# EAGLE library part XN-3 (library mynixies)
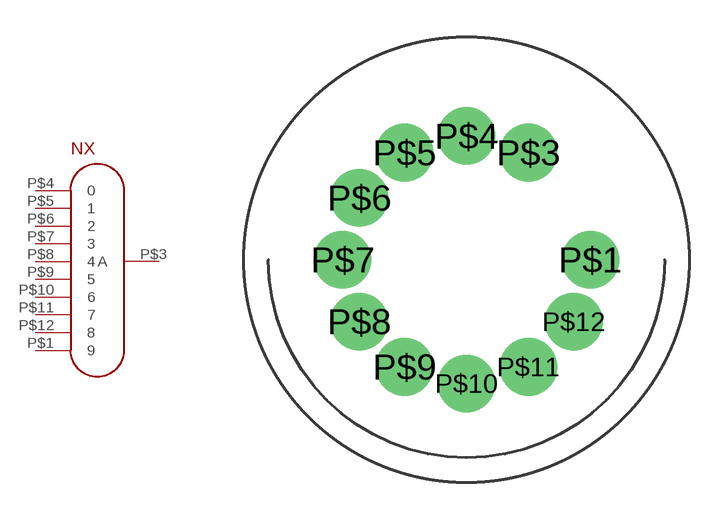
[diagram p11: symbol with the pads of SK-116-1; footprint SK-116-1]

Designator prefix NX

## XN-3  [SK-116-1]
P$1  9
P$3  A
P$4  0
P$5  1
P$6  2
P$7  3
P$8  4
P$9  5
P$10  6
P$11  7
P$12  8

## Footprint SK-116-1 (pad centres in mm)
drill 1.55: P$1 5,0; P$3 2.5,4.33; P$4 0,5; P$5 -2.5,4.33; P$6 -4.33,2.5; P$7 -5,0; P$8 -4.33,-2.5; P$9 -2.5,-4.33; P$10 0,-5; P$11 2.5,-4.33; P$12 4.33,-2.5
